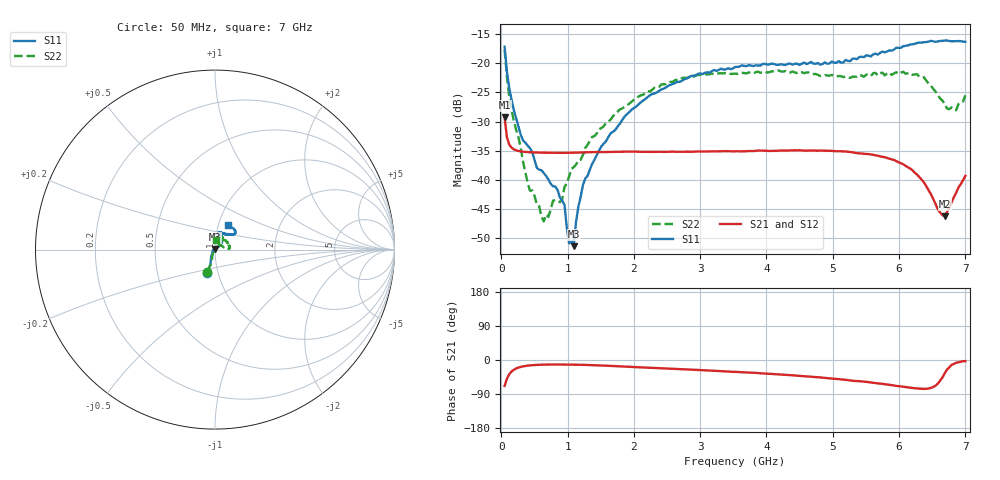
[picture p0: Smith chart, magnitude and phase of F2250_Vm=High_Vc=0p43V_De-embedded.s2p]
! Integrated Device Technology
! Corporate Headquarters
! 6024 Silver Creek Valley Road
! San Jose, CA 95138  USA
! Phone:  1-408-284-8200
! Toll Free:  1-800-223-1366
! Webpage:  http://www.idt.com/
! Timing and RF Division
! 515 Groton Road, Suite 102
! Westford, MA 01886-6024
! Device:  F2250
! Description: Voltage Variable RF Attenuator
! Frequency:  50.0 -  6000.00 MHz
! Package:  3x3 mm Thin QFN Plastic Package: 16 pin
! Ports:  2 RF, 3 DC
!  Pin  1  = GND
!  Pin  2  = NC
!  Pin  3  = RF1  = Port 1
!  Pin  4  = NC
!  Pin  5  = GND
!  Pin  6  = GND
!  Pin  7  = GND
!  Pin  8  = GND
!  Pin  9  = NC
!  Pin 10  = RF2  = Port 2
!  Pin 11  = NC
!  Pin 12  = GND
!  Pin 13  = GND
!  Pin 14  = VCNTRL
!  Pin 15  = VDD
!  Pin 16  = VMODE
! Vcntrl:  0.430 Volts
! Vmode:  +3.300 Volts
! Vdd:  +3.30  Volts
! Current:  1.264 mA
! Data:  The device was measured on a the F2250 evaluation board which has
!  individual transmission lines to the RF pins.  Data was collected
!  using a calibrated network analyzer.  The evaluation board was
!  de-embedded using a TRL calibration technique.
!  The reference plane is the edge of the package pin.
! Misc:  SN 10
!  Action Tracker AT0258
! Date Measured:  2014-11-26
! Date:  2015-10-15  MJV
! Note:
!  Integrated Device Technology supplies this data as a sample of measured
!  data at the package pin for this product.  Your particular data for this
!  product may vary.
!  Data was taken at 25 degrees C.
!  Integrated Device Technology reserves the right to change this data at anytime.
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# GHz S dB R 50
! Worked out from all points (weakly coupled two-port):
!   201 points, 50 MHz to 7 GHz, reference 50 ohm
!   highest |S21| = -29.30 dB at 50 MHz (marker M1); lowest = -46.2 dB at 6.687 GHz (marker M2)
!   lowest |S11| = -51.3 dB at 1.093 GHz (marker M3), VSWR 1.01, Z = 50 + j0.271 ohm
!   |S11| at or under -10 dB: start of sweep to end of sweep
!   |S22| runs from -47.1 to -17.7 dB; largest |S21 - S12| = 5.8e-05
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0.05  -17.18 -108.5  -29.30 -68.5  -29.29 -68.5  -17.70 -108.9
0.1195  -24.20 -111.9  -33.91 -37.6  -33.91 -37.6  -25.65 -108.2
0.29325  -32.26 -127.4  -35.11 -18.2  -35.11 -18.2  -34.47 -117.7
0.43225  -34.55 -145.3  -35.26 -14.2  -35.26 -14.2  -41.84 -152.9
0.5365  -37.92 -154.7  -35.31 -12.9  -35.30 -12.9  -44.24 -172.3
0.64075  -38.81 -162.6  -35.33 -12.2  -35.33 -12.2  -47.10 142.9
0.77975  -41.09 176.2  -35.35 -11.9  -35.35 -11.9  -43.56 112.1
0.91875  -43.51 156.2  -35.36 -11.9  -35.35 -11.9  -43.32 87.4
0.9535  -44.28 170.6  -35.35 -11.9  -35.36 -11.9  -41.20 91.6
1.023  -50.88 140.6  -35.35 -12.0  -35.34 -12.1  -39.41 74.2
1.0925  -51.35 90.3  -35.33 -12.2  -35.33 -12.2  -37.78 68.5
1.12725  -47.19 60.6  -35.32 -12.3  -35.32 -12.3  -37.36 61.9
1.2315  -40.85 40.5  -35.28 -12.7  -35.28 -12.7  -35.70 51.4
1.6485  -32.02 41.0  -35.20 -15.5  -35.21 -15.5  -29.67 47.4
2.37825  -24.75 46.6  -35.17 -21.5  -35.17 -21.5  -24.08 47.4
3.525  -20.65 71.7  -35.10 -31.3  -35.10 -31.3  -21.78 69.5
4.7065  -20.06 72.0  -34.95 -44.7  -34.95 -44.6  -21.86 68.4
5.85325  -17.79 40.5  -36.35 -65.4  -36.35 -65.6  -21.60 20.1
6.3745  -16.40 40.9  -40.42 -76.2  -40.42 -76.2  -22.39 3.8
6.68725  -16.11 47.8  -46.22 -35.3  -46.21 -35.1  -26.94 25.7
6.861  -16.22 54.5  -42.20 -7.4  -42.16 -7.5  -28.04 58.2
7  -16.33 62.4  -39.30 -3.0  -39.27 -3.2  -25.50 86.5
